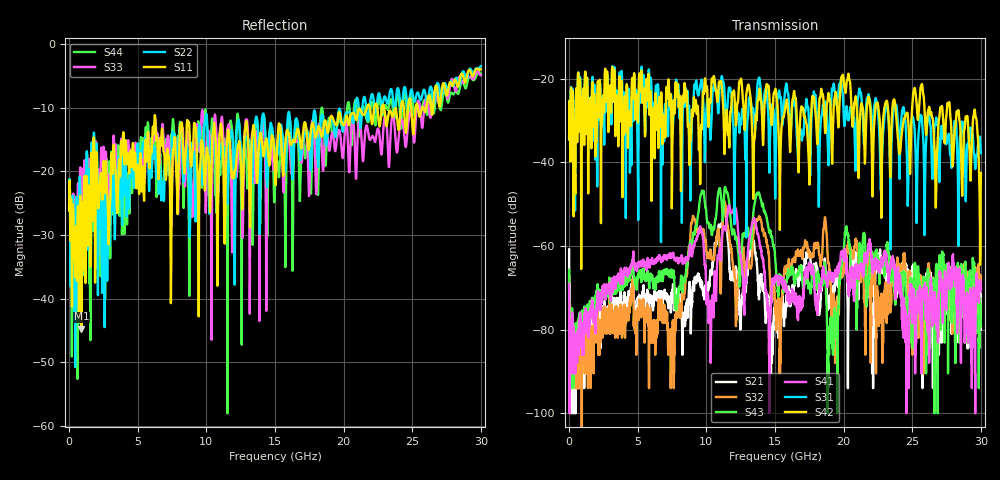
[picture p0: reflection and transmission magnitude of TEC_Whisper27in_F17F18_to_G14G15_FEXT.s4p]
! Tyco Electronics
! F17F18-G14G15_FEXT
!! PART DESCRIPTION: Whisper 27in Megtron 6 VLP-HVLP-VLP Channel Model, bulkhead 2.4mm test pts
!! MODEL DESCRIPTION: System 4-port S-parameter
!! MODEL STATUS: Measured
!! MODEL GEOMETRY: Channel Model
!! MODEL FREQUENCY RANGE: DC to 30.000 GHz in 10.000 MHz frequency steps
!! MODEL EDGE RATE LIMITATION: 12.500 ps (Using conservative 0.5/Fmax rule of thumb)
!! TIME-DOMAIN TRANSFORM CAUTIONS:
!! 1.) Do not simulate transient edge rates faster than the number listed above.  Edge rates faster than this number
!!  contain significant spectral content at frequencies above the model's highest frequency.
!! 2.) Even when simulating edge rates that are slower than the number listed above, be aware that the best time
!!  resolution possible with a direct iFFT is (1 / 2Fmax).  As a result, time resolution is typically not adequate
!!  for most time-domain simulations unless tricks such as windowing are used to minimize leakage and aliasing.
!! 3.) Because the model has a uniform frequency step, a direct iFFT will result in an impulse that that has a time
!!  length given by either (1 / Fstep) or (1 / 2Fstep), depending on the transform being used.  Care has been taken
!!  in selecting the frequency step to ensure a settled impulse response for the model.  Therefore, convolution with
!!  the model's impulse response should present no issues.  However, if directly concatenating s-parameter models
!!  in the frequency domain a user must either interpolate necessary interim frequencies or complete impulse response
!!  zero-padding.  Impulse response zero-padding is more difficult, but more accurate.
!! PORT DEFINITIONS:
!! Port  1  ----->  Side A  F17  G14  Side B  <-----  Port  2
!! Port  3  ----->  Side A  F18  G15  Side B  <-----  Port  4
! Point-to-Point link (differential)  !
! Connectors:  !
!  1: STRADA Whisper  !
! Materials:  !
!  Backplane: Megtron-6 HVLP  !
!  Daughtercard: Megtron-6 VLP  !
! Stack-up:  !
!  Backplane: 20 layers, 200mil thick  !
!  Daughtercard: 14 layers, 110mil thick  !
! Trace Length:  !
!  Backplane: 17in  !
!  Daightercards: 5in  !
! Trace Width:  !
!  Backplane: 8-13-8 mils  !
!  Daughtercards: 6-9-6 mils  !
! Geometry:  !
!  Backplane: Stripline  !
!  Daughtercards: Stripline  !
! Freq. Range: 0 GHz - 30 GHz  !
! Note1: non-mixed-mode s-parameters  !
! Note2: channel includes 2.4mm test points  !
! Touchstone data converted from IdEM dataset
# GHz S MA R 50
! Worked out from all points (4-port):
!   3000 points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, 10 MHz to 30 GHz, reference 50 ohm
!   strongest paths, dB at 10 MHz, 7.51 GHz, 15.01 GHz, 22.51 GHz, 30 GHz:
!     S42: -34.5, -40.8, -22.7, -26.3, -42.6
!     S31: -34.5, -31.1, -46.7, -28.0, -37.8
!     S41: -69.1, -62.3, -68.2, -64.9, -70.2
!     S43: -65.7, -66.0, -62.7, -63.5, -79.2
!     S32: -67.3, -81.9, -74.0, -75.4, -67.3
!     S21: -60.8, -71.4, -73.2, -64.4, -80.0
!   lowest |S11| = -44.8 dB at 910 MHz (marker M1), VSWR 1.01, Z = 50.5 - j0.228 ohm
!   |S11| at or under -10 dB: start of sweep to 21.7 GHz; 22.45 GHz to 22.8 GHz (342.1 MHz wide, 1.51 % of centre); 22.96 GHz to 24.17 GHz (1.211 GHz wide, 5.14 % of centre)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
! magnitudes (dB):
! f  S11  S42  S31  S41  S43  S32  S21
! 10 MHz  -26.1  -34.5  -34.5  -69.1  -65.7  -67.3  -60.8
! 910 MHz  -44.8  -38.0  -34.1  -84.4  -80.0  -88.0  -86.0
! 9.55 GHz  -19.4  -45.0  -21.7  -55.3  -48.6  -56.4  -68.9
! 10.29 GHz  -25.6  -25.3  -34.6  -74.9  -55.1  -60.8  -66.7
! 11.45 GHz  -17.5  -28.3  -28.9  -55.2  -46.8  -52.4  -53.3
! 14.76 GHz  -14.5  -31.1  -26.4  -70.8  -57.8  -71.1  -86.0
! 30 GHz  -3.9  -42.6  -37.8  -70.2  -79.2  -67.3  -80.0
